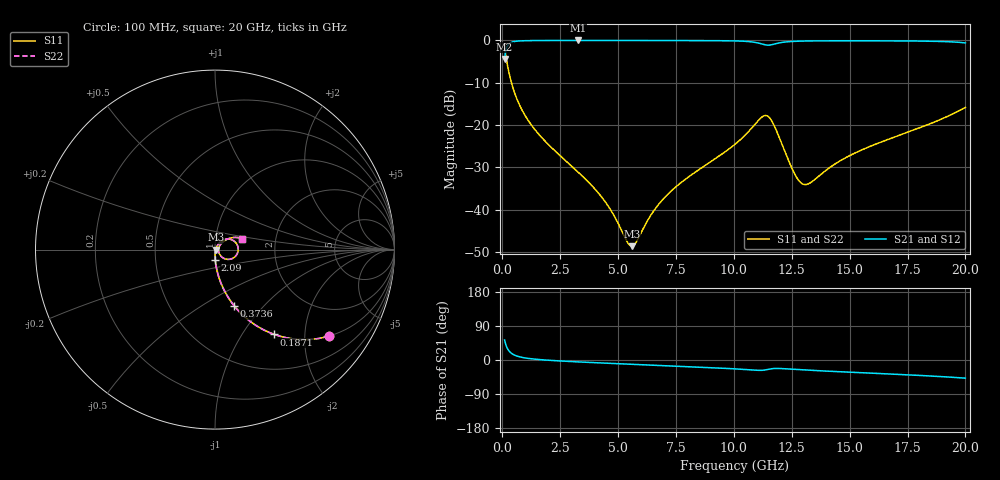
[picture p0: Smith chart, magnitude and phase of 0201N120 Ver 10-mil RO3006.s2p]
# GHz S MA R 50
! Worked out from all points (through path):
!   1601 points, 100 MHz to 20 GHz, reference 50 ohm
!   highest |S21| = -0.03 dB at 3.272 GHz (marker M1); lowest = -4.4 dB at 100 MHz (marker M2)
!   group delay of S21, straight-line fit = 7.28 ps
!   lowest |S11| = -48.6 dB at 5.597 GHz (marker M3), VSWR 1.01, Z = 50.4 - j0.0842 ohm
!   |S11| at or under -10 dB: 394.6 MHz to end of sweep
!   |S22| runs from -48.6 to -2.0 dB; largest |S21 - S12| = 0
!   S11 on the Smith chart (normalised r, x): 100 MHz: 0.99, -2.63; 187.1 MHz: 0.99, -1.41; 373.6 MHz: 0.99, -0.70; 2.09 GHz: 1.00, -0.11; 20 GHz: 1.34, +0.17
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0.1  0.7972 -37.3  0.6029 52.7  0.6029 52.7  0.7972 -37.3
0.1870625  0.5764 -55.1  0.8161 34.8  0.8161 34.8  0.5764 -55.1
0.274125  0.4334 -64.7  0.9001 25.1  0.9001 25.1  0.4334 -64.7
0.373625  0.3322 -71.2  0.9421 18.6  0.9421 18.6  0.3322 -71.2
0.9955  0.1279 -84.0  0.9902 5.3  0.9902 5.3  0.1279 -84.0
2.09  0.05526 -88.8  0.9963 -1.1  0.9963 -1.1  0.05526 -88.8
3.271562  0.02787 -89.4  0.9968 -5.0  0.9968 -5.0  0.02787 -89.4
3.420812  0.0255 -89.2  0.9968 -5.4  0.9968 -5.4  0.0255 -89.2
4.453125  0.01228 -83.1  0.9966 -8.3  0.9966 -8.3  0.01228 -83.1
5.597375  0.003699 -13.1  0.9962 -11.3  0.9962 -11.3  0.003699 -13.1
6.741625  0.01145 53.9  0.9955 -14.2  0.9955 -14.2  0.01145 53.9
7.736625  0.02104 59.6  0.9946 -16.7  0.9946 -16.7  0.02104 59.6
10.05  0.05914 53.3  0.9845 -23.4  0.9845 -23.4  0.05914 53.3
10.97038  0.1063 31.6  0.9405 -27.1  0.9405 -27.1  0.1063 31.6
11.443  0.128 -6.1  0.878 -25.3  0.878 -25.3  0.128 -6.1
11.7415  0.09848 -33.1  0.9028 -22.4  0.9028 -22.4  0.09848 -33.1
12.74894  0.02315 -28.1  0.9766 -25.3  0.9766 -25.3  0.02315 -28.1
13.035  0.01982 -5.9  0.9811 -26.3  0.9811 -26.3  0.01982 -5.9
13.37081  0.02135 16.4  0.9842 -27.4  0.9842 -27.4  0.02135 16.4
14.75137  0.03998 42.6  0.9879 -31.5  0.9879 -31.5  0.03998 42.6
16.69162  0.06802 43.5  0.9859 -36.8  0.9859 -36.8  0.06802 43.5
20  0.1613 21.9  0.9321 -47.9  0.9321 -47.9  0.1613 21.9
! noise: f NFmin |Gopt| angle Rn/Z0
0.1  0.0007118  0.9396  0.3495  0.00263
2.301  0.004534  0.7974  4.717  0.004624
4.515  0.007586  0.767  9.123  0.006582
6.729  0.01061  0.7545  13.51  0.008611
8.943  0.0155  0.7751  17.86  0.01374
11.14  0.06058  0.9228  22.25  0.1673
13.36  0.02827  0.8144  26.56  0.03016
15.57  0.02519  0.7657  30.73  0.02034
17.79  0.03105  0.7829  34.88  0.02676
20  0.06632  0.8807  39.09  0.1069
